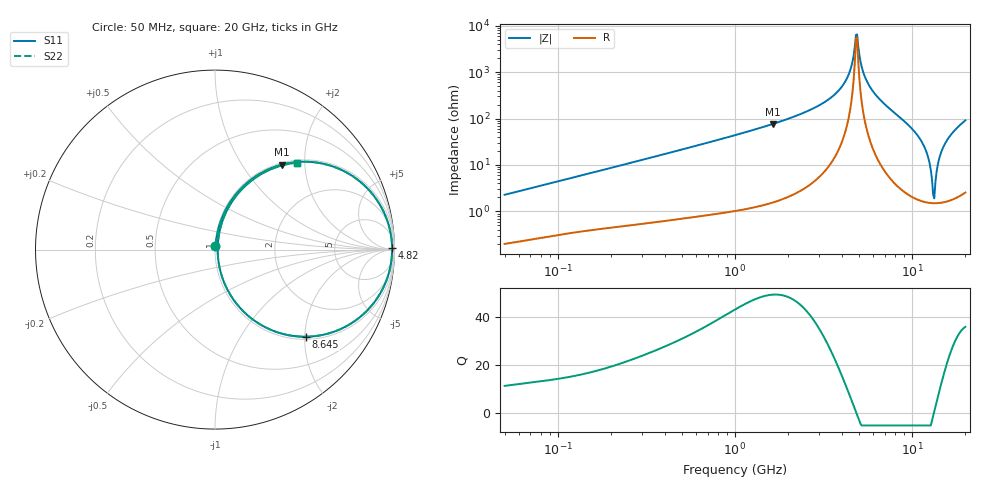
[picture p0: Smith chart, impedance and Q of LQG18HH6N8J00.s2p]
!Murata Part Number: LQG18HH6N8J00
!These Parameters are Measured in Series Mode Connection
!  o--[Z]--o
!Port1  Port2
!  o-------o
!Freq. Start=50[MHz] Stop=20[GHz], 401[Steps]
# Hz S RI R 50
!Freq.(Hz) S11(Real) S11(Imag) S21(Real) S21(Imag) S12(Real) S12(Imag) S22(Real) S22(Imag)
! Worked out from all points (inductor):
!   401 points, 50 MHz to 20 GHz, reference 50 ohm
!   read as one part in series: L = 7.16 nH near 51.52 MHz
!   highest Q = 49.1 at 1.639 GHz (marker M1), where L = 7.43 nH
!   self-resonance near 4.82 GHz
!   S11 on the Smith chart (normalised r, x): 50 MHz: 1.00, +0.05; 4.82 GHz: open; 8.645 GHz: 1.06, -2.02; 20 GHz: 1.05, +1.83
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5e7  0.0025 0.0226  0.9975 -0.0226  0.9975 -0.0226  0.0025 0.0226
1.364002e8  0.0072 0.0591  0.9928 -0.0591  0.9928 -0.0591  0.0072 0.0591
3.721004e8  0.0303 0.1537  0.9697 -0.1537  0.9697 -0.1537  0.0303 0.1537
1e9  0.1663 0.3609  0.8337 -0.3609  0.8337 -0.3609  0.1663 0.3609
1.639343e9  0.3722 0.4733  0.6278 -0.4733  0.6278 -0.4733  0.3722 0.4733
2.728004e9  0.7159 0.4385  0.2841 -0.4385  0.2841 -0.4385  0.7159 0.4385
3.466789e9  0.8761 0.3109  0.1239 -0.3109  0.1239 -0.3109  0.8761 0.3109
4.087748e9  0.9547 0.1755  0.0453 -0.1755  0.0453 -0.1755  0.9547 0.1755
4.472136e9  0.9792 0.0876  0.0208 -0.0876  0.0208 -0.0876  0.9792 0.0876
4.81993e9  0.9868 0.00856  0.0132 -0.00856  0.0132 -0.00856  0.9868 0.00856
4.966507e9  0.9862 -0.0242  0.0138 0.0242  0.0138 0.0242  0.9862 -0.0242
5.194772e9  0.981 -0.074  0.019 0.074  0.019 0.074  0.981 -0.074
5.598765e9  0.9601 -0.1578  0.0399 0.1578  0.0399 0.1578  0.9601 -0.1578
7.442007e9  0.7241 -0.431  0.2759 0.431  0.2759 0.431  0.7241 -0.431
8.644534e9  0.5059 -0.4854  0.4941 0.4854  0.4941 0.4854  0.5059 -0.4854
1.149051e10  0.0887 -0.2573  0.9113 0.2573  0.9113 0.2573  0.0887 -0.2573
1.220001e10  0.0406 -0.1559  0.9594 0.1559  0.9594 0.1559  0.0406 -0.1559
1.295331e10  0.0169 -0.0453  0.9831 0.0453  0.9831 0.0453  0.0169 -0.0453
1.334722e10  0.0149 0.0114  0.9851 -0.0114  0.9851 -0.0114  0.0149 0.0114
1.417136e10  0.0305 0.1229  0.9695 -0.1229  0.9695 -0.1229  0.0305 0.1229
1.527346e10  0.084 0.2502  0.916 -0.2502  0.916 -0.2502  0.084 0.2502
2e10  0.4558 0.4843  0.5442 -0.4843  0.5442 -0.4843  0.4558 0.4843
